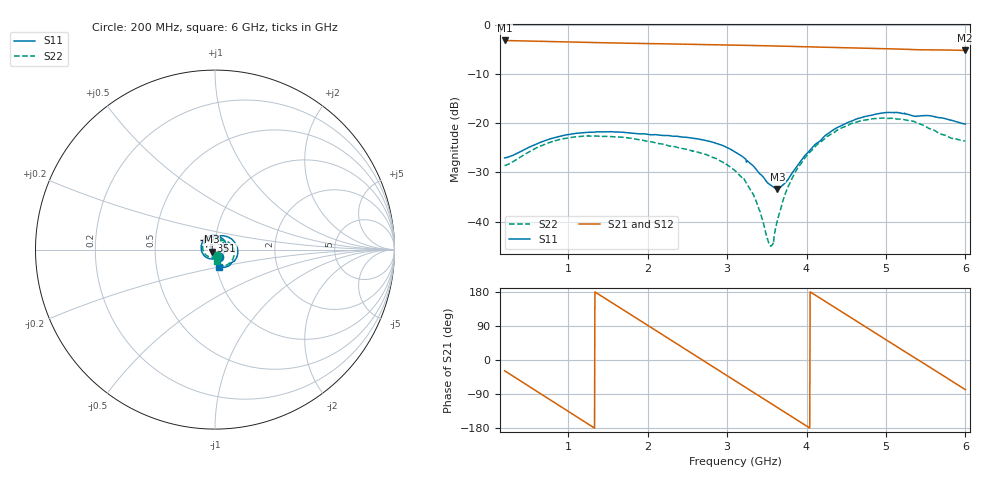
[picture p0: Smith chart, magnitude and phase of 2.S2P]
!Agilent Technologies,E5071C,MY46316741,A.11.02
!Date: Fri Apr 15 16:19:41 2022
!Data & Calibration Information:
!Freq	S11:SOLT2(ON)	S21:SOLT2(ON)	S12:SOLT2(ON)	S22:SOLT2(ON)
!PortZ  Port1:50+j0  Port2:50+j0
!Above PortZ is port z conversion or system Z0 setting when saving the data.
!When reading, reference impedance value at option line is always used.
# Hz S dB R 50
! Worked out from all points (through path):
!   1200 points, 200 MHz to 6 GHz, reference 50 ohm
!   highest |S21| = -3.19 dB at 200 MHz (marker M1); lowest = -5.2 dB at 5.995 GHz (marker M2)
!   group delay of S21, straight-line fit = 369 ps
!   lowest |S11| = -33.3 dB at 3.635 GHz (marker M3), VSWR 1.04, Z = 48.2 - j1.14 ohm
!   |S11| at or under -10 dB: start of sweep to end of sweep
!   |S22| runs from -45.0 to -18.9 dB; largest |S21 - S12| = 0.0021
!   S11 on the Smith chart (normalised r, x): 200 MHz: 1.04, -0.08; 1.351 GHz: 0.88, +0.09; 6 GHz: 1.03, -0.20
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2e8  -27.04 -63.1  -3.19 -28.4  -3.19 -28.4  -28.60 -74.3
4.563803e8  -25.30 -106.3  -3.30 -62.6  -3.30 -62.7  -26.28 -118.8
6.788991e8  -23.71 -139.2  -3.38 -92.5  -3.38 -92.5  -24.46 -152.5
9.062552e8  -22.61 -169.0  -3.46 -122.9  -3.46 -122.9  -23.28 176.9
1.167473e9  -21.97 160.7  -3.55 -157.8  -3.55 -157.8  -22.67 145.2
1.351293e9  -21.77 141.3  -3.62 177.7  -3.62 177.7  -22.59 124.8
1.781818e9  -21.97 100.6  -3.76 120.6  -3.76 120.6  -23.03 81.3
2.134946e9  -22.37 71.9  -3.85 73.7  -3.85 73.8  -24.12 50.2
2.401001e9  -22.73 49.0  -3.92 38.4  -3.92 38.4  -25.04 29.2
2.628357e9  -23.18 28.2  -3.99 8.1  -3.99 8.2  -25.87 11.2
2.855713e9  -24.05 5.1  -4.05 -22.1  -4.06 -22.1  -27.13 -8.9
3.102419e9  -25.85 -24.2  -4.13 -54.9  -4.14 -54.9  -29.66 -34.0
3.33945e9  -28.83 -60.6  -4.22 -86.4  -4.22 -86.4  -34.75 -65.8
3.537781e9  -32.43 -111.1  -4.29 -112.8  -4.29 -112.7  -44.73 -149.2
3.634529e9  -33.34 -146.6  -4.32 -125.7  -4.32 -125.6  -39.62 137.2
3.813511e9  -30.27 151.3  -4.40 -149.4  -4.40 -149.3  -31.36 96.7
4.069892e9  -25.01 100.2  -4.51 176.6  -4.51 176.7  -25.42 63.8
4.582652e9  -19.46 36.1  -4.70 108.7  -4.70 108.8  -19.98 9.1
5.037364e9  -17.82 -10.2  -4.89 48.7  -4.89 48.8  -19.02 -35.2
5.496914e9  -18.44 -45.3  -5.09 -11.7  -5.09 -11.6  -20.64 -70.7
5.995163e9  -20.15 -75.9  -5.21 -77.7  -5.22 -77.6  -23.61 -79.4
6e9  -20.16 -75.9  -5.21 -78.3  -5.23 -78.3  -23.62 -79.0
